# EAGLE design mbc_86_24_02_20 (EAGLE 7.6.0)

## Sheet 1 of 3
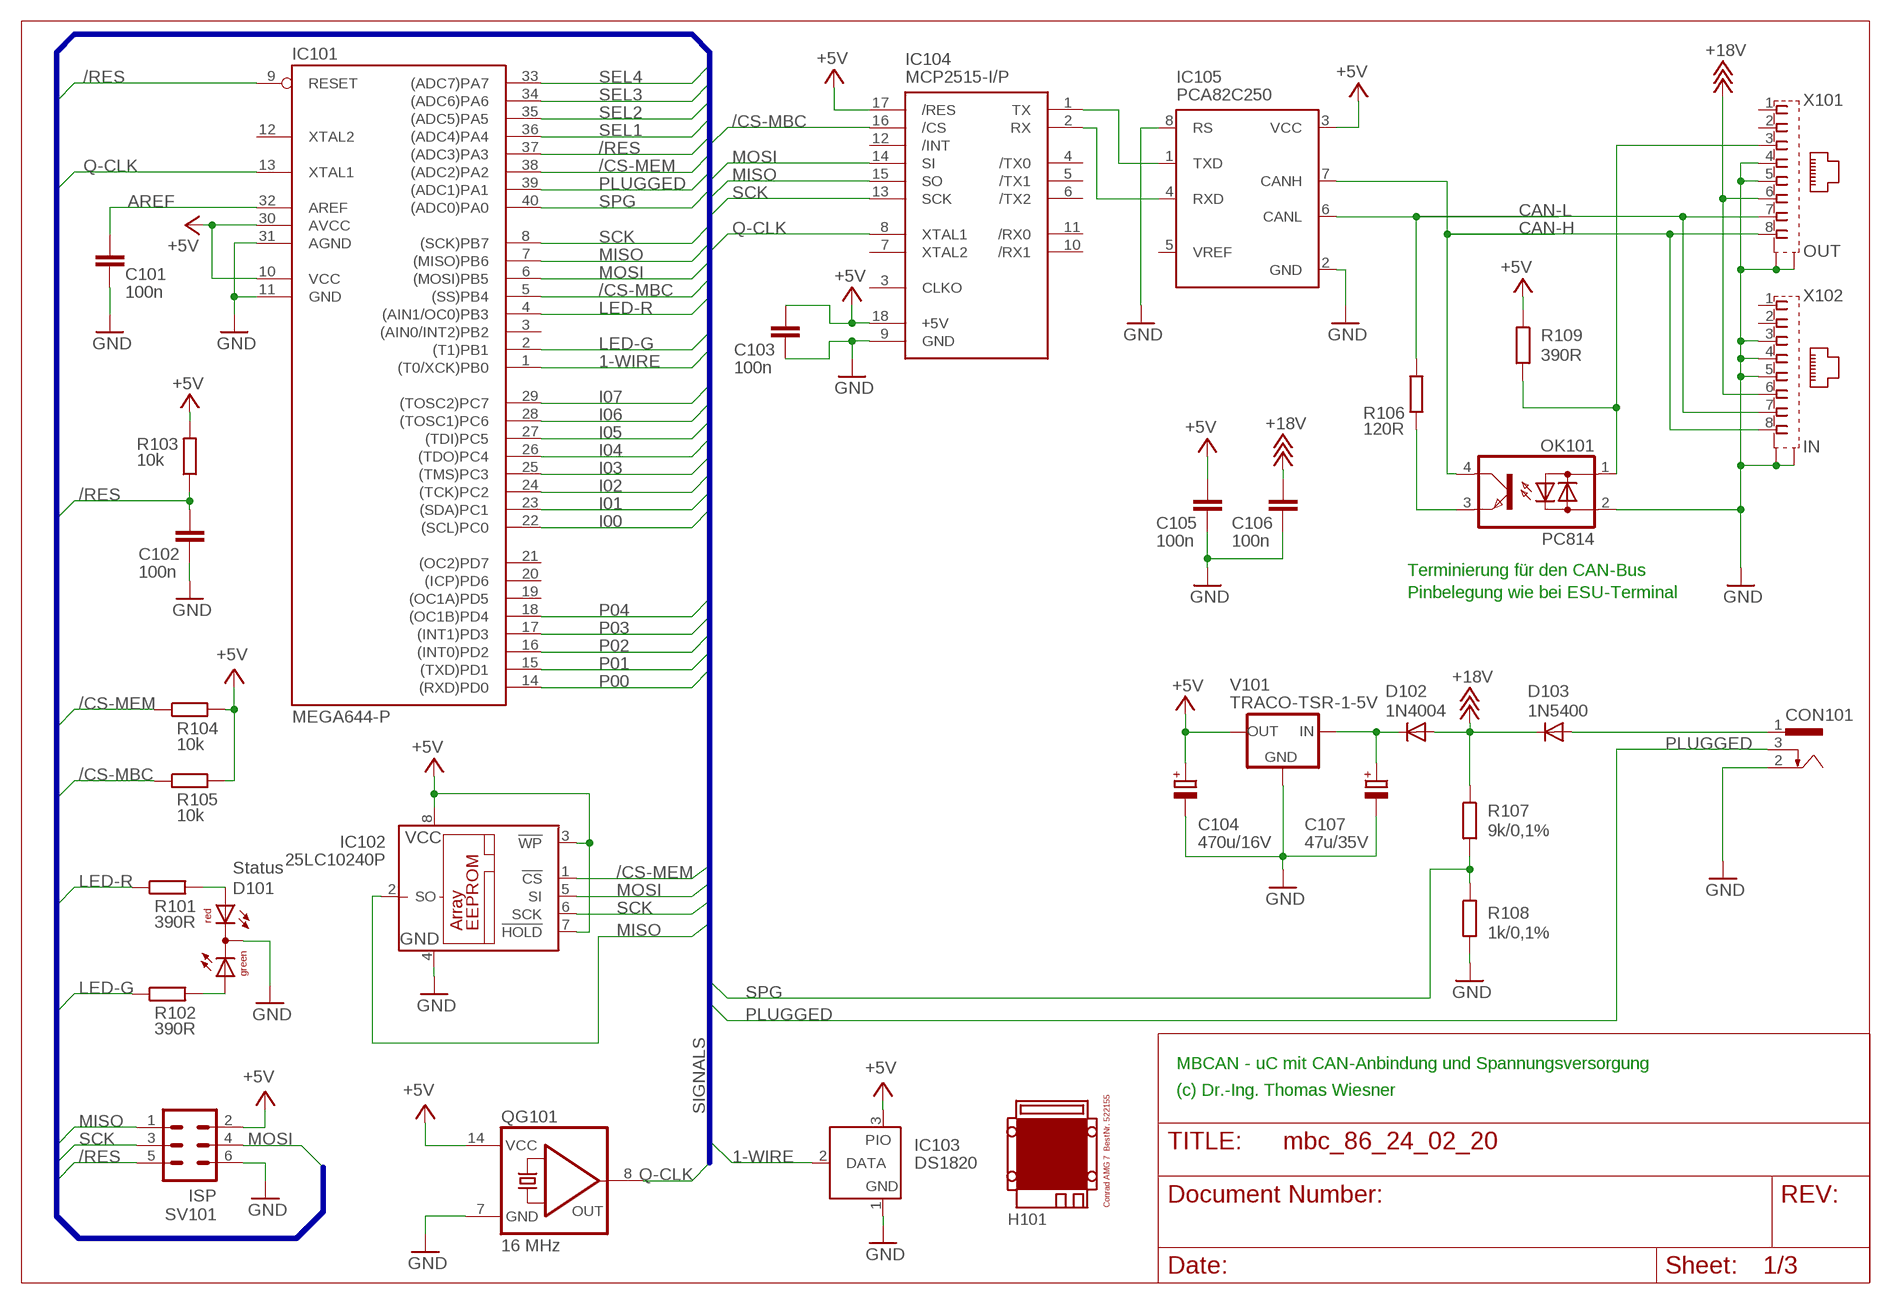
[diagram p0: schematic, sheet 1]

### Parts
C101  100n  C-EU025-025X050  [C025-025X050]
C102  100n  C-EU025-025X050  [C025-025X050]
C103  100n  C-EU025-025X050  [C025-025X050]
C104  470u/16V  CPOL-EUE3.5-8  [E3,5-8]
C105  100n  C-EU025-025X050  [C025-025X050]
C106  100n  C-EU025-025X050  [C025-025X050]
C107  47u/35V  CPOL-EUE2.5-7  [E2,5-7]
CON101  POWER-JACK  [POWER-JACK]
D101  Status  DUOLED5MM  [DUOLED5MM]
D102  1N4004  [DO41-10]
D103  1N5400  [DO201-15]
H101  MODULGEHÄUSE-AMG-7  [MODULGEHÄUSE-AMG-7]
IC101  MEGA644-P  MEGA323-P  [DIL40]
IC102  25LC10240P  25LC040P  [DIL8]
IC103  DS1820  DS2405  [TO92-]
IC104  MCP2515-I/P  MCP2510-I/P  [DIL18]
IC105  PCA82C250  [DIL08]
OK101  PC814  [DIL04]
QG101  16 MHz  QG5860  [DIL14S]
R101  390R  R-EU_0207/10  [0207/10]
R102  390R  R-EU_0207/10  [0207/10]
R103  10k  R-EU_0207/10  [0207/10]
R104  10k  R-EU_0207/10  [0207/10]
R105  10k  R-EU_0207/10  [0207/10]
R106  120R  R-EU_0207/10  [0207/10]
R107  9k/0,1%  R-EU_0207/10  [0207/10]
R108  1k/0,1%  R-EU_0207/10  [0207/10]
R109  390R  R-EU_0207/10  [0207/10]
SV101  ISP  ML6  [ML6]
V101  TRACO-TSR-1-5V  [TRACO-TSR-1]
X101  OUT  0446200002  [0446200002]
X102  IN  0446200002  [0446200002]

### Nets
1-WIRE: IC101.1((T0/XCK)PB0) IC103.2(DATA)
+5V: C103.1 C104.+ C105.1 IC101.10(VCC) IC101.30(AVCC) IC102.3(!WP) IC102.7(!HOLD) IC102.8(VCC) IC103.3(PIO) IC104.17(/RES) IC104.18(+5V) IC105.3(VCC) QG101.14(VCC) R103.2 R104.2 R105.2 R109.1 SV101.2 V101.OUT ; also sheet 2,3
+18V: C106.1 D102.A D103.C R107.1 X101.6 X102.6 ; also sheet 2
/CS-MBC: IC101.5((SS)PB4) IC104.16(/CS) R105.1
/CS-MEM: IC101.38((ADC2)PA2) IC102.1(!CS) R104.1
/RES: C102.1 IC101.9(RESET) IC101.37((ADC3)PA3) R103.1 SV101.5
AREF: C101.1 IC101.32(AREF)
CAN-H: IC105.7(CANH) OK101.4(C) X101.8 X102.8
CAN-L: IC105.6(CANL) R106.2 X101.7 X102.7
GND: C101.2 C102.2 C103.2 C104.- C105.2 C106.2 C107.- CON101.2 D101.K(C) IC101.11(GND) IC101.31(AGND) IC102.4(GND) IC103.1(GND) IC104.9(GND) IC105.2(GND) IC105.8(RS) OK101.2(AC2) QG101.7(GND) R108.2 SV101.6 V101.GND X101.4 X101.5 X101.S@1(S1) X101.S@2(S2) X102.3 X102.4 X102.5 X102.S@1(S1) X102.S@2(S2) ; also sheet 2,3
I00: IC101.22((SCL)PC0) ; also sheet 3
I01: IC101.23((SDA)PC1) ; also sheet 3
I02: IC101.24((TCK)PC2) ; also sheet 3
I03: IC101.25((TMS)PC3) ; also sheet 3
I04: IC101.26((TDO)PC4) ; also sheet 3
I05: IC101.27((TDI)PC5) ; also sheet 3
I06: IC101.28((TOSC1)PC6) ; also sheet 3
I07: IC101.29((TOSC2)PC7) ; also sheet 3
LED-G: IC101.2((T1)PB1) R102.1
LED-R: IC101.4((AIN1/OC0)PB3) R101.1
MISO: IC101.7((MISO)PB6) IC102.2(SO) IC104.15(SO) SV101.1
MOSI: IC101.6((MOSI)PB5) IC102.5(SI) IC104.14(SI) SV101.4
N$1: IC104.1(TX) IC105.1(TXD)
N$2: IC104.2(RX) IC105.4(RXD)
N$3: OK101.3(E) R106.1
N$5: OK101.1(AC1) R109.2 X101.3
N$6: C107.+ D102.C V101.IN
N$9: D101.AR R101.2
N$13: D101.AG R102.2
P00: IC101.14((RXD)PD0) ; also sheet 2
P01: IC101.15((TXD)PD1) ; also sheet 2
P02: IC101.16((INT0)PD2) ; also sheet 2
P03: IC101.17((INT1)PD3) ; also sheet 2
P04: IC101.18((OC1B)PD4) ; also sheet 2
PLUGGED: CON101.3 IC101.39((ADC1)PA1)
Q-CLK: IC101.13(XTAL1) IC104.8(XTAL1) QG101.8(OUT)
SCK: IC101.8((SCK)PB7) IC102.6(SCK) IC104.13(SCK) SV101.3
SEL1: IC101.36((ADC4)PA4) ; also sheet 2
SEL2: IC101.35((ADC5)PA5) ; also sheet 2
SEL3: IC101.34((ADC6)PA6)
SEL4: IC101.33((ADC7)PA7)
SPG: IC101.40((ADC0)PA0) R107.2 R108.1
V-NETZTEIL1: CON101.1 D103.A
Unconnected: IC101.3((AIN0/INT2)PB2) IC101.12(XTAL2) IC101.19((OC1A)PD5) IC101.20((ICP)PD6) IC101.21((OC2)PD7) IC104.3(CLKO) IC104.4(/TX0) IC104.5(/TX1) IC104.6(/TX2) IC104.7(XTAL2) IC104.10(/RX1) IC104.11(/RX0) IC104.12(/INT) IC105.5(VREF) X101.1 X101.2 X102.1 X102.2

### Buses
SIGNALS

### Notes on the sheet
- Terminierung für den CAN-Bus
- Pinbelegung wie bei ESU-Terminal
- MBCAN - uC mit CAN-Anbindung und Spannungsversorgung
- (c) Dr.-Ing. Thomas Wiesner

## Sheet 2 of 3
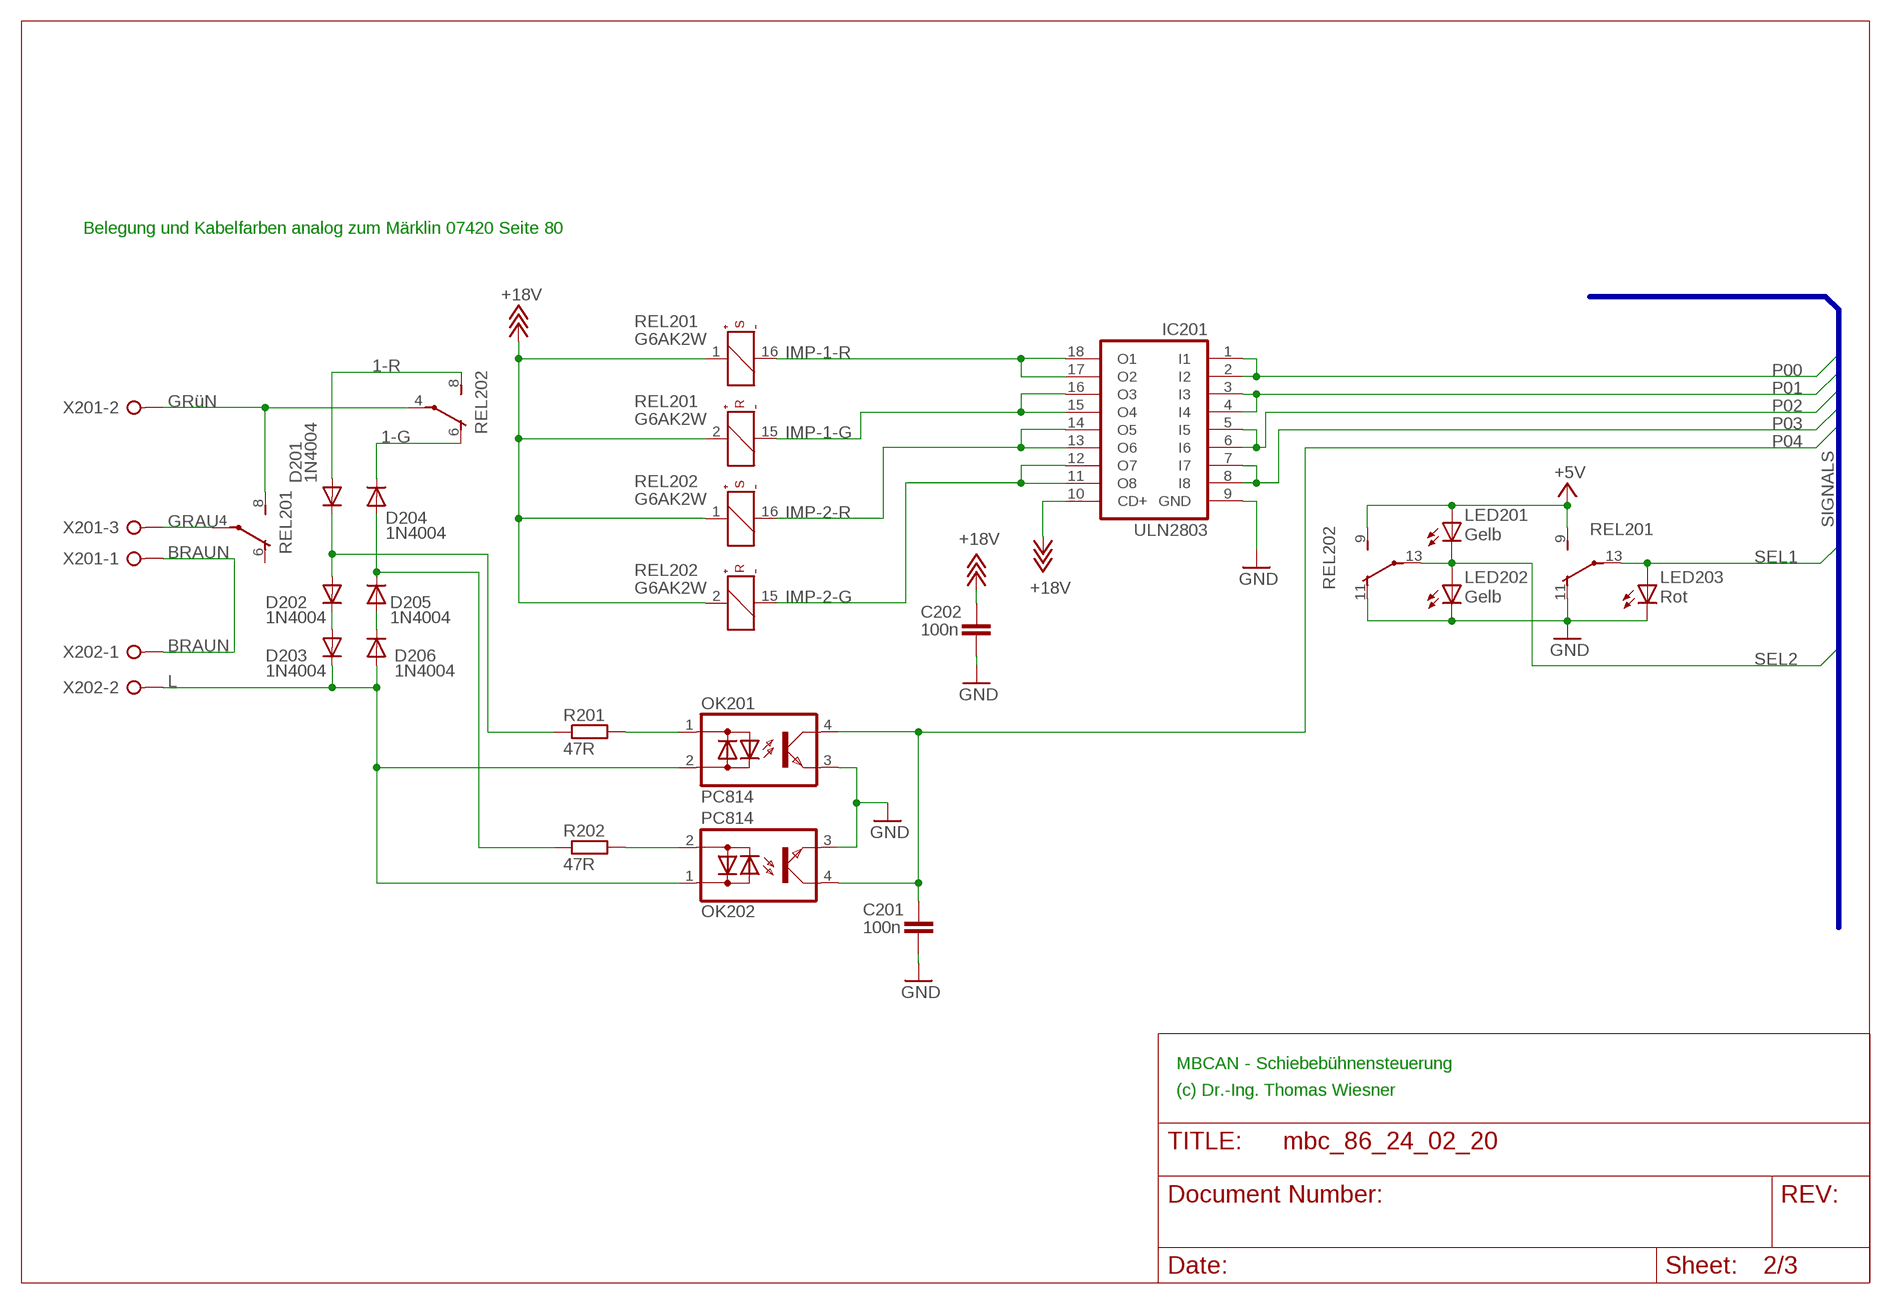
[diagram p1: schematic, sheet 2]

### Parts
C201  100n  C-EU025-025X050  [C025-025X050]
C202  100n  C-EU025-025X050  [C025-025X050]
D201  1N4004  [DO41-10]
D202  1N4004  [DO41-10]
D203  1N4004  [DO41-10]
D204  1N4004  [DO41-10]
D205  1N4004  [DO41-10]
D206  1N4004  [DO41-10]
IC201  ULN2803  ULN2803A  [DIL18]
LED201  Gelb  LED3MM  [LED3MM]
LED202  Gelb  LED3MM  [LED3MM]
LED203  Rot  LED3MM  [LED3MM]
OK201  PC814  [DIL04]
OK202  PC814  [DIL04]
R201  47R  R-EU_0207/10  [0207/10]
R202  47R  R-EU_0207/10  [0207/10]
REL201  G6AK2W  [REL-BIPOLAR]
REL202  G6AK2W  [REL-BIPOLAR]
X201  W237-03P  [W237-133]
X202  W237-02P  [W237-132]

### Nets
1-G: D204.C REL202.6(O)
1-R: D201.A REL202.8(S)
+5V: LED201.A REL201.9(S) REL202.9(S) ; also sheet 1,3
+18V: C202.1 IC201.10(CD+) REL201.1(+) REL201.2(+) REL202.1(+) REL202.2(+) ; also sheet 1
BRAUN: X201.1 X202.1
GND: C201.2 C202.2 IC201.9(GND) LED202.K(C) LED203.K(C) OK201.3(E) OK202.3(E) REL201.11(O) REL202.11(O) ; also sheet 1,3
GRAU: REL201.4(P) X201.3
GRüN: REL201.8(S) REL202.4(P) X201.2
IMP-1-G: IC201.15(O4) IC201.16(O3) REL201.15(-)
IMP-1-R: IC201.17(O2) IC201.18(O1) REL201.16(-)
IMP-2-G: IC201.11(O8) IC201.12(O7) REL202.15(-)
IMP-2-R: IC201.13(O6) IC201.14(O5) REL202.16(-)
L: D203.C D206.A OK201.2(AC2) OK202.1(AC1) X202.2
N$4: D202.C D203.A
N$7: D205.A D206.C
N$8: OK202.2(AC2) R202.2
N$10: OK201.1(AC1) R201.2
P00: IC201.1(I1) IC201.2(I2) ; also sheet 1
P01: IC201.3(I3) IC201.4(I4) ; also sheet 1
P02: IC201.5(I5) IC201.6(I6) ; also sheet 1
P03: IC201.7(I7) IC201.8(I8) ; also sheet 1
P04: C201.1 OK201.4(C) OK202.4(C) ; also sheet 1
SCH-1-G: D204.A D205.C R202.1
SCH-1-R: D201.C D202.A R201.1
SEL1: LED203.A REL201.13(P) ; also sheet 1
SEL2: LED201.K(C) LED202.A REL202.13(P) ; also sheet 1
Unconnected: REL201.6(O)

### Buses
SIGNALS

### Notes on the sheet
- Belegung und Kabelfarben analog zum Märklin 07420 Seite 80
- MBCAN - Schiebebühnensteuerung
- (c) Dr.-Ing. Thomas Wiesner

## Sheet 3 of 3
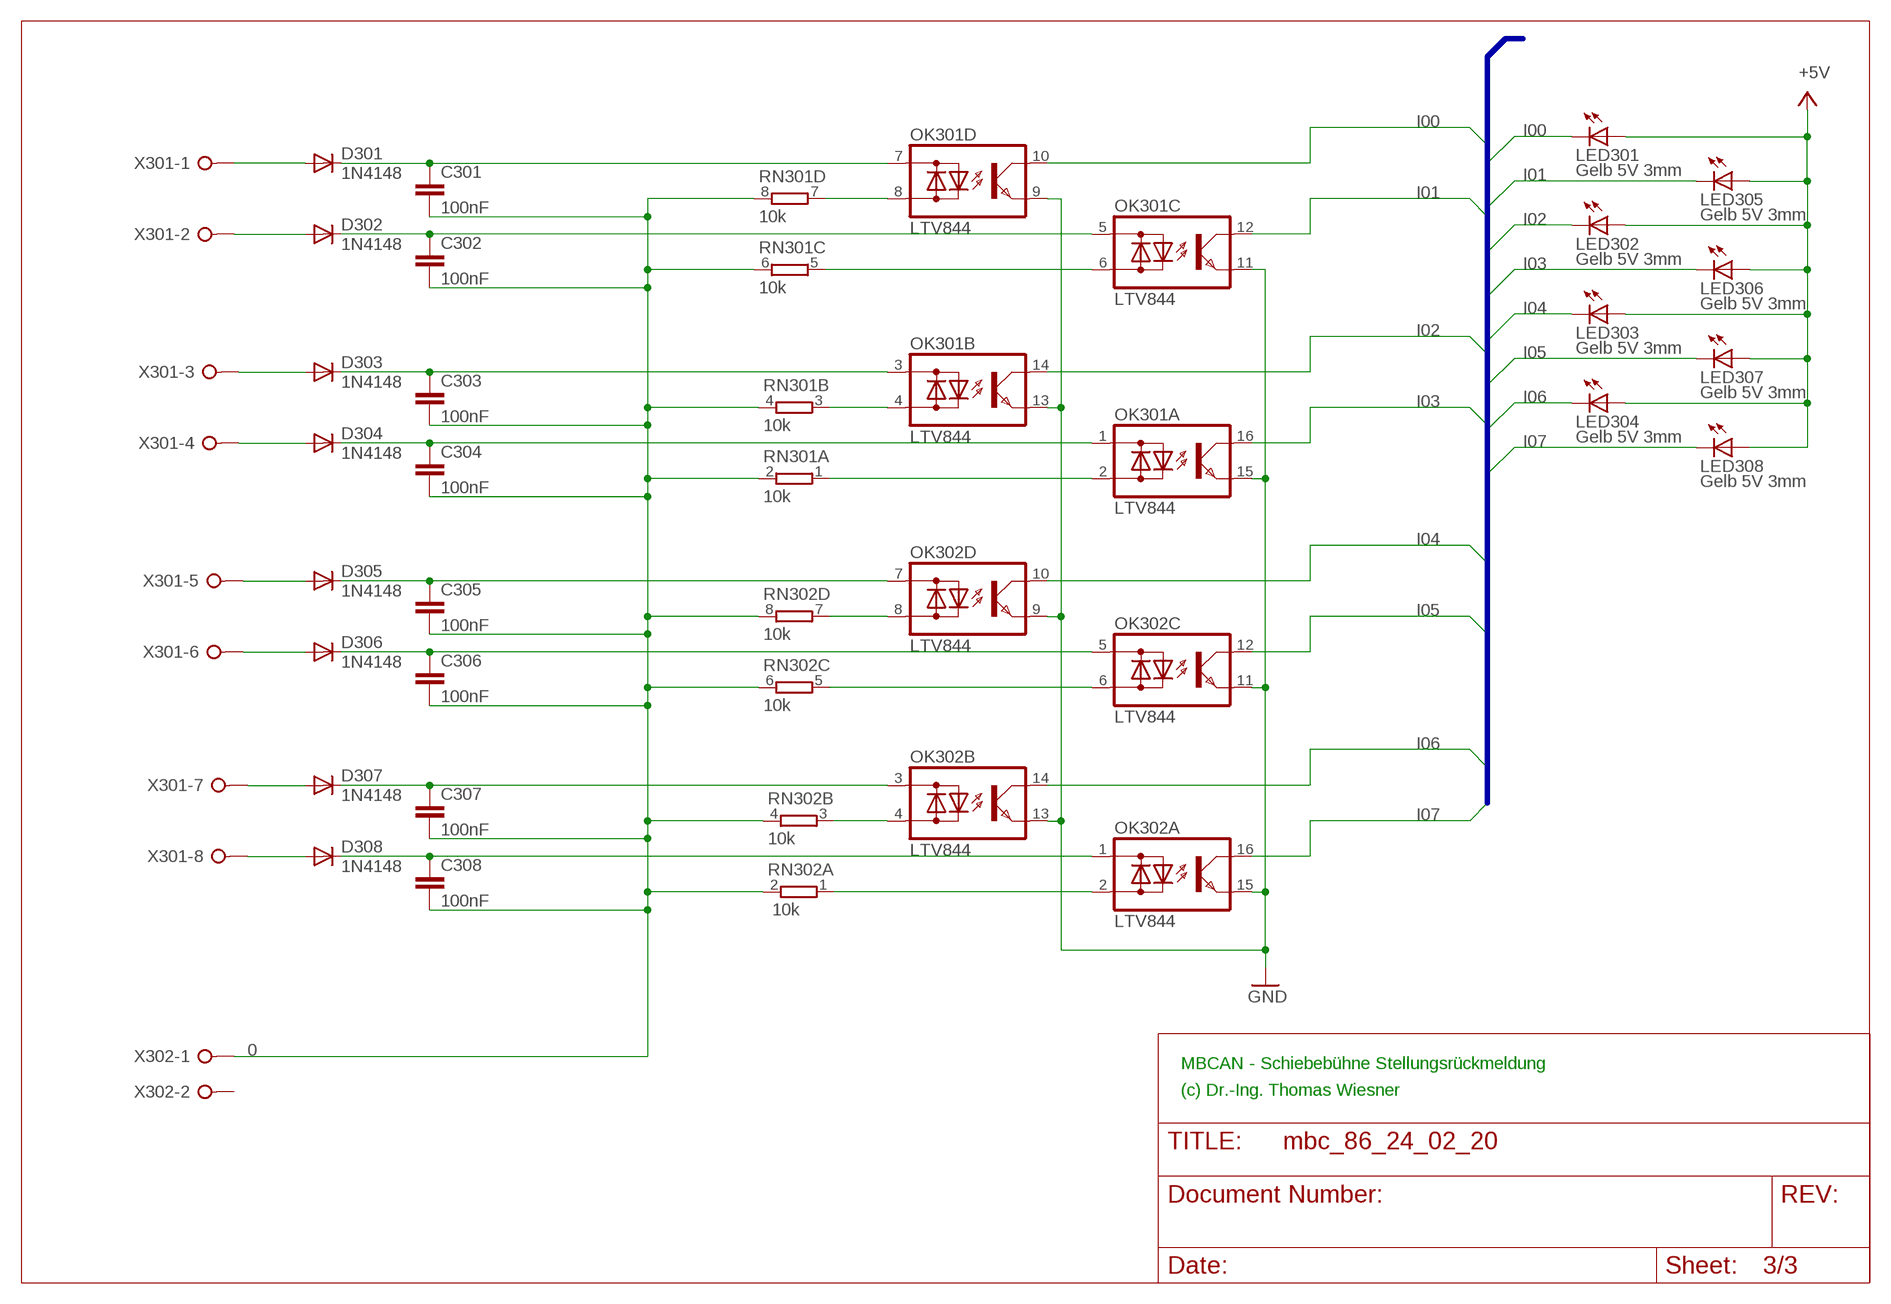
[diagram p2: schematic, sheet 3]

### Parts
C301  100nF  C-EU025-025X050  [C025-025X050]
C302  100nF  C-EU025-025X050  [C025-025X050]
C303  100nF  C-EU025-025X050  [C025-025X050]
C304  100nF  C-EU025-025X050  [C025-025X050]
C305  100nF  C-EU025-025X050  [C025-025X050]
C306  100nF  C-EU025-025X050  [C025-025X050]
C307  100nF  C-EU025-025X050  [C025-025X050]
C308  100nF  C-EU025-025X050  [C025-025X050]
D301  1N4148  1N4148DO35-10  [DO35-10]
D302  1N4148  1N4148DO35-10  [DO35-10]
D303  1N4148  1N4148DO35-10  [DO35-10]
D304  1N4148  1N4148DO35-10  [DO35-10]
D305  1N4148  1N4148DO35-10  [DO35-10]
D306  1N4148  1N4148DO35-10  [DO35-10]
D307  1N4148  1N4148DO35-10  [DO35-10]
D308  1N4148  1N4148DO35-10  [DO35-10]
LED301  Gelb 5V 3mm  LED3MM  [LED3MM]
LED302  Gelb 5V 3mm  LED3MM  [LED3MM]
LED303  Gelb 5V 3mm  LED3MM  [LED3MM]
LED304  Gelb 5V 3mm  LED3MM  [LED3MM]
LED305  Gelb 5V 3mm  LED3MM  [LED3MM]
LED306  Gelb 5V 3mm  LED3MM  [LED3MM]
LED307  Gelb 5V 3mm  LED3MM  [LED3MM]
LED308  Gelb 5V 3mm  LED3MM  [LED3MM]
OK301  LTV844  TIL196  [DIL16]
OK302  LTV844  TIL196  [DIL16]
RN301  10k  E4R  [SIL8]
RN302  10k  E4R  [SIL8]
X301  W237-08P  [W237-8P]
X302  W237-02P  [W237-132]

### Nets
0: C301.2 C302.2 C303.2 C304.2 C305.2 C306.2 C307.2 C308.2 RN301.2 RN301.4 RN301.6 RN301.8 RN302.2 RN302.4 RN302.6 RN302.8 X302.1
+5V: LED301.A LED302.A LED303.A LED304.A LED305.A LED306.A LED307.A LED308.A ; also sheet 1,2
GND: OK301.9(D:E) OK301.11(C:E) OK301.13(B:E) OK301.15(A:E) OK302.9(D:E) OK302.11(C:E) OK302.13(B:E) OK302.15(A:E) ; also sheet 1,2
I00: LED301.K(C) OK301.10(D:C) ; also sheet 1
I01: LED305.K(C) OK301.12(C:C) ; also sheet 1
I02: LED302.K(C) OK301.14(B:C) ; also sheet 1
I03: LED306.K(C) OK301.16(A:C) ; also sheet 1
I04: LED303.K(C) OK302.10(D:C) ; also sheet 1
I05: LED307.K(C) OK302.12(C:C) ; also sheet 1
I06: LED304.K(C) OK302.14(B:C) ; also sheet 1
I07: LED308.K(C) OK302.16(A:C) ; also sheet 1
N$11: D301.A X301.1
N$12: C301.1 D301.C OK301.7(D:AC1)
N$14: C302.1 D302.C OK301.5(C:AC1)
N$15: C303.1 D303.C OK301.3(B:AC1)
N$16: D302.A X301.2
N$17: D303.A X301.3
N$18: C304.1 D304.C OK301.1(A:AC1)
N$19: D304.A X301.4
N$20: C305.1 D305.C OK302.7(D:AC1)
N$21: C306.1 D306.C OK302.5(C:AC1)
N$22: C307.1 D307.C OK302.3(B:AC1)
N$23: C308.1 D308.C OK302.1(A:AC1)
N$24: D305.A X301.5
N$25: D306.A X301.6
N$26: D308.A X301.8
N$27: D307.A X301.7
N$42: OK302.2(A:AC2) RN302.1
N$43: OK302.4(B:AC2) RN302.3
N$44: OK302.6(C:AC2) RN302.5
N$45: OK302.8(D:AC2) RN302.7
N$46: OK301.2(A:AC2) RN301.1
N$48: OK301.4(B:AC2) RN301.3
N$64: OK301.6(C:AC2) RN301.5
N$65: OK301.8(D:AC2) RN301.7
Unconnected: X302.2

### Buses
B$1

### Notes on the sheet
- MBCAN - Schiebebühne Stellungsrückmeldung
- (c) Dr.-Ing. Thomas Wiesner

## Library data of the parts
C101-C103 C105 C106 C201 C202 C301-C308 = rcl:C-EU: CAPACITOR, European symbol
C104 C107 = rcl:CPOL-EU: POLARIZED CAPACITOR, European symbol
CON101 = mbc:POWER-JACK: Power-Stecker für 2,5 mm Hohlbuchse
D101 = led:DUOLED5MM: DUO LED 2 colors, 5 mm, round
D102 D201-D206 = diode:1N4004: DIODE
D103 = diode:1N5400: DIODE
D301-D308 = diode:1N4148: DIODE
H101 = mbc:MODULGEHÄUSE-AMG-7: Gehäuse
IC101 = atmel:MEGA323-P: MICROCONTROLLER 32 Kbytes FLASH 2 Kbytes SRAM 1 Kbytes EEPROM USART 8-channel 10 bit ADC Source: avr.lbr; OC_FARNELL: unknown; OC_NEWARK: unknown
IC102 = microchip:25*: Serial EEPROM 4K/ 8K , SPI bus; MF: MICROCHIP; MPN: 25LC040/P; OC_FARNELL: 9758100; OC_NEWARK: 96K4091
IC103 = maxim:DS2405: Addressable Switch DALLAS Semiconductor; MF: DALLAS SEMICONDUCTOR; MPN: DS2405; OC_FARNELL: 1188025; OC_NEWARK: 06F4645
IC104 = mbc:MCP2510: BASIC-CAN 2.0a Controller Stand-alone CAN controller von Microchip
IC105 = micro-philips:PCA82C250: CAN CONTROLLER INTERFACE; OC_FARNELL: 3692358; OC_NEWARK: unknown
IC201 = uln-udn:ULN2803A: DRIVER ARRAY
LED201-LED203 LED301-LED308 = led:LED: LED
OK101 OK201 OK202 = optocoupler:PC814: SHARP OPTO COUPLER; OC_FARNELL: 9707662; OC_NEWARK: unknown
OK301 OK302 = optocoupler:TIL196: TEXAS INSTRUMENTS OPTO COUPLER; MPN: TIL 196; OC_FARNELL: 1683367; OC_NEWARK: 05R6476
QG101 = crystal:QG5860: CRYSTAL RESONATOR; OC_FARNELL: unknown; OC_NEWARK: unknown
R101-R109 = resistor:R-EU_: RESISTOR, European symbol
R201 R202 = rcl:R-EU_: RESISTOR, European symbol
REL201 REL202 = mbc:G6AK2W: Bipolares Relais 2xUM 12V
RN301 RN302 = resistor-sil:E4R: SIL RESISTOR; OC_FARNELL: unknown; OC_NEWARK: unknown
SV101 = con-ml:ML6: HARTING; OC_FARNELL: unknown; OC_NEWARK: unknown
V101 = mbc:TRACO-TSR-1-5V: Spannungsregler Hersteller: TRACO Typ: TSR-1 5V: TSR 1-2450 Spg: 5V Strom: 1A Reichelt TSR 1-2450
X101 X102 = mbc:0446200002: RJ-45 INVERTED MODULAR JACK ASSEMBLY WITH RJ-11 KEEPOUT FEATURE Source: Data sheet MOLEX 0446200002 BUCHSE, RJ45, GESCHIRMT Source: Farnell; MF: MOLEX; MPN: 0446200002; OC_FARNELL: 9251910
X201 = con-wago-508:W237-03P: WAGO SREW CLAMP; OC_FARNELL: unknown; OC_NEWARK: unknown
X202 X302 = con-wago-508:W237-02P: WAGO SREW CLAMP; OC_FARNELL: unknown; OC_NEWARK: unknown
X301 = con-wago-508:W237-08P: WAGO SREW CLAMP; OC_FARNELL: unknown; OC_NEWARK: unknown

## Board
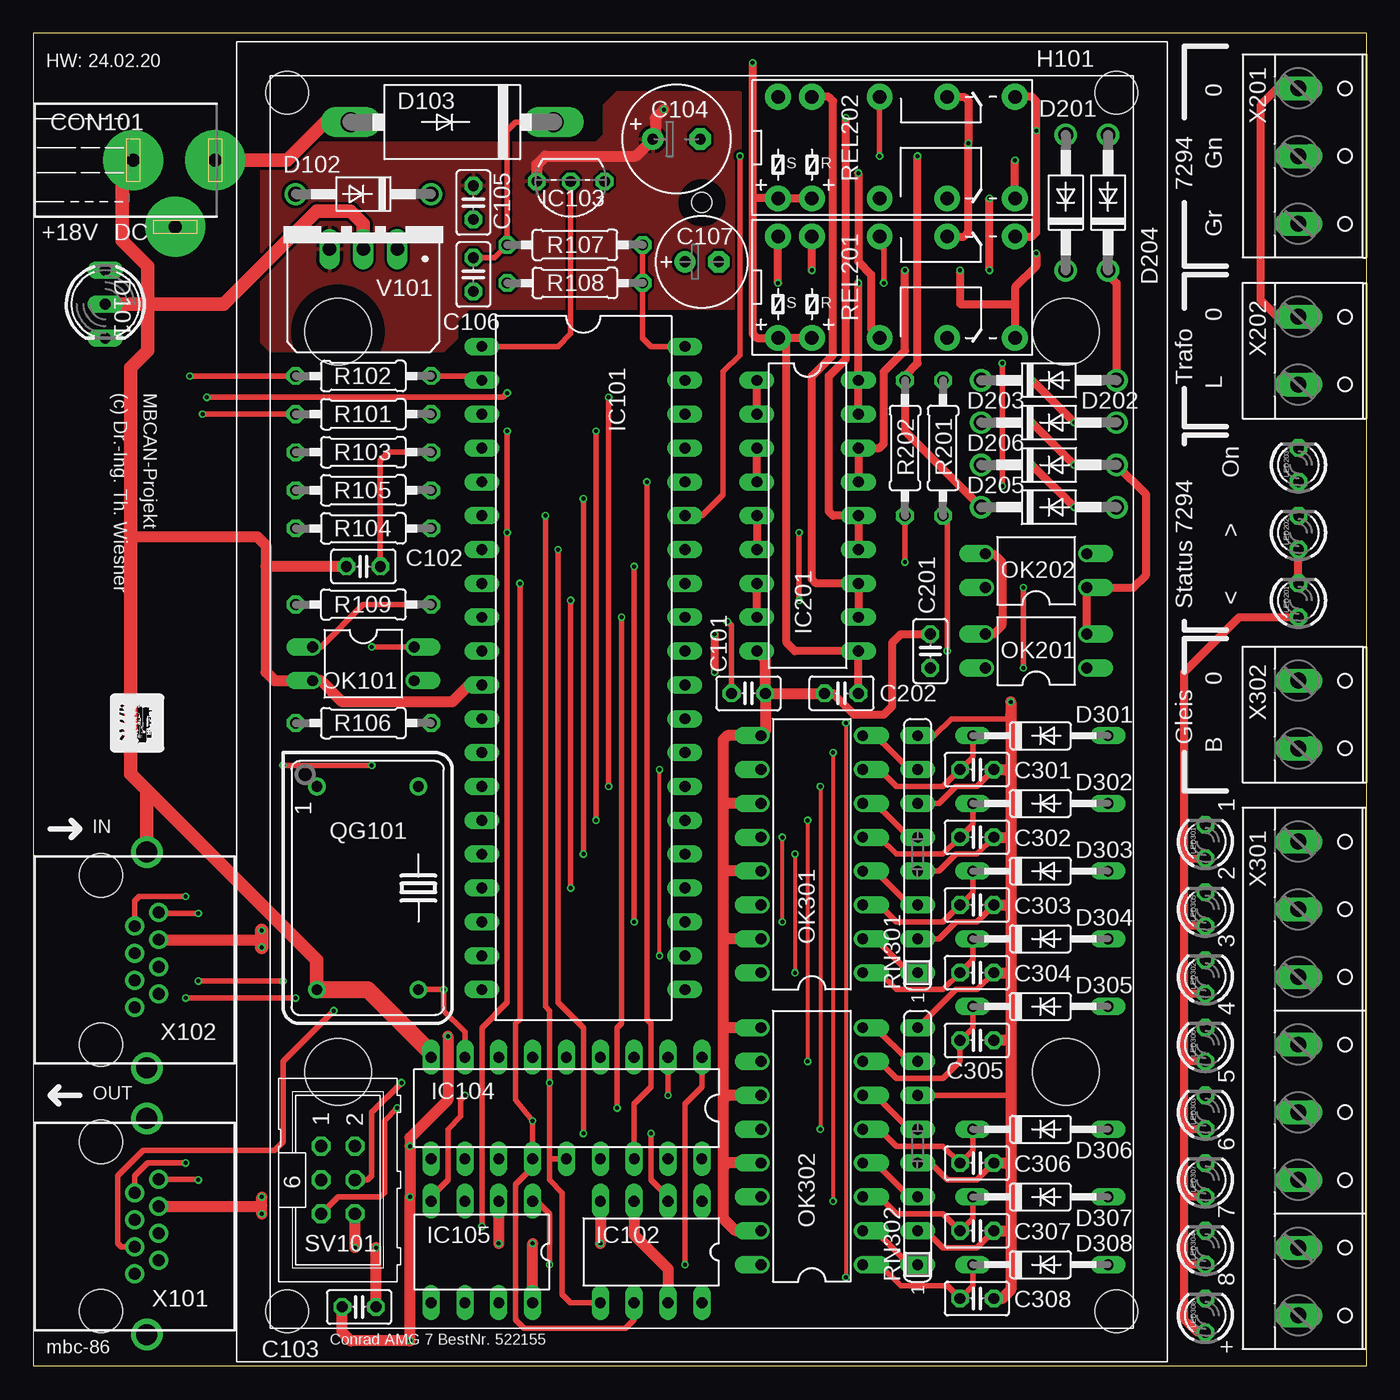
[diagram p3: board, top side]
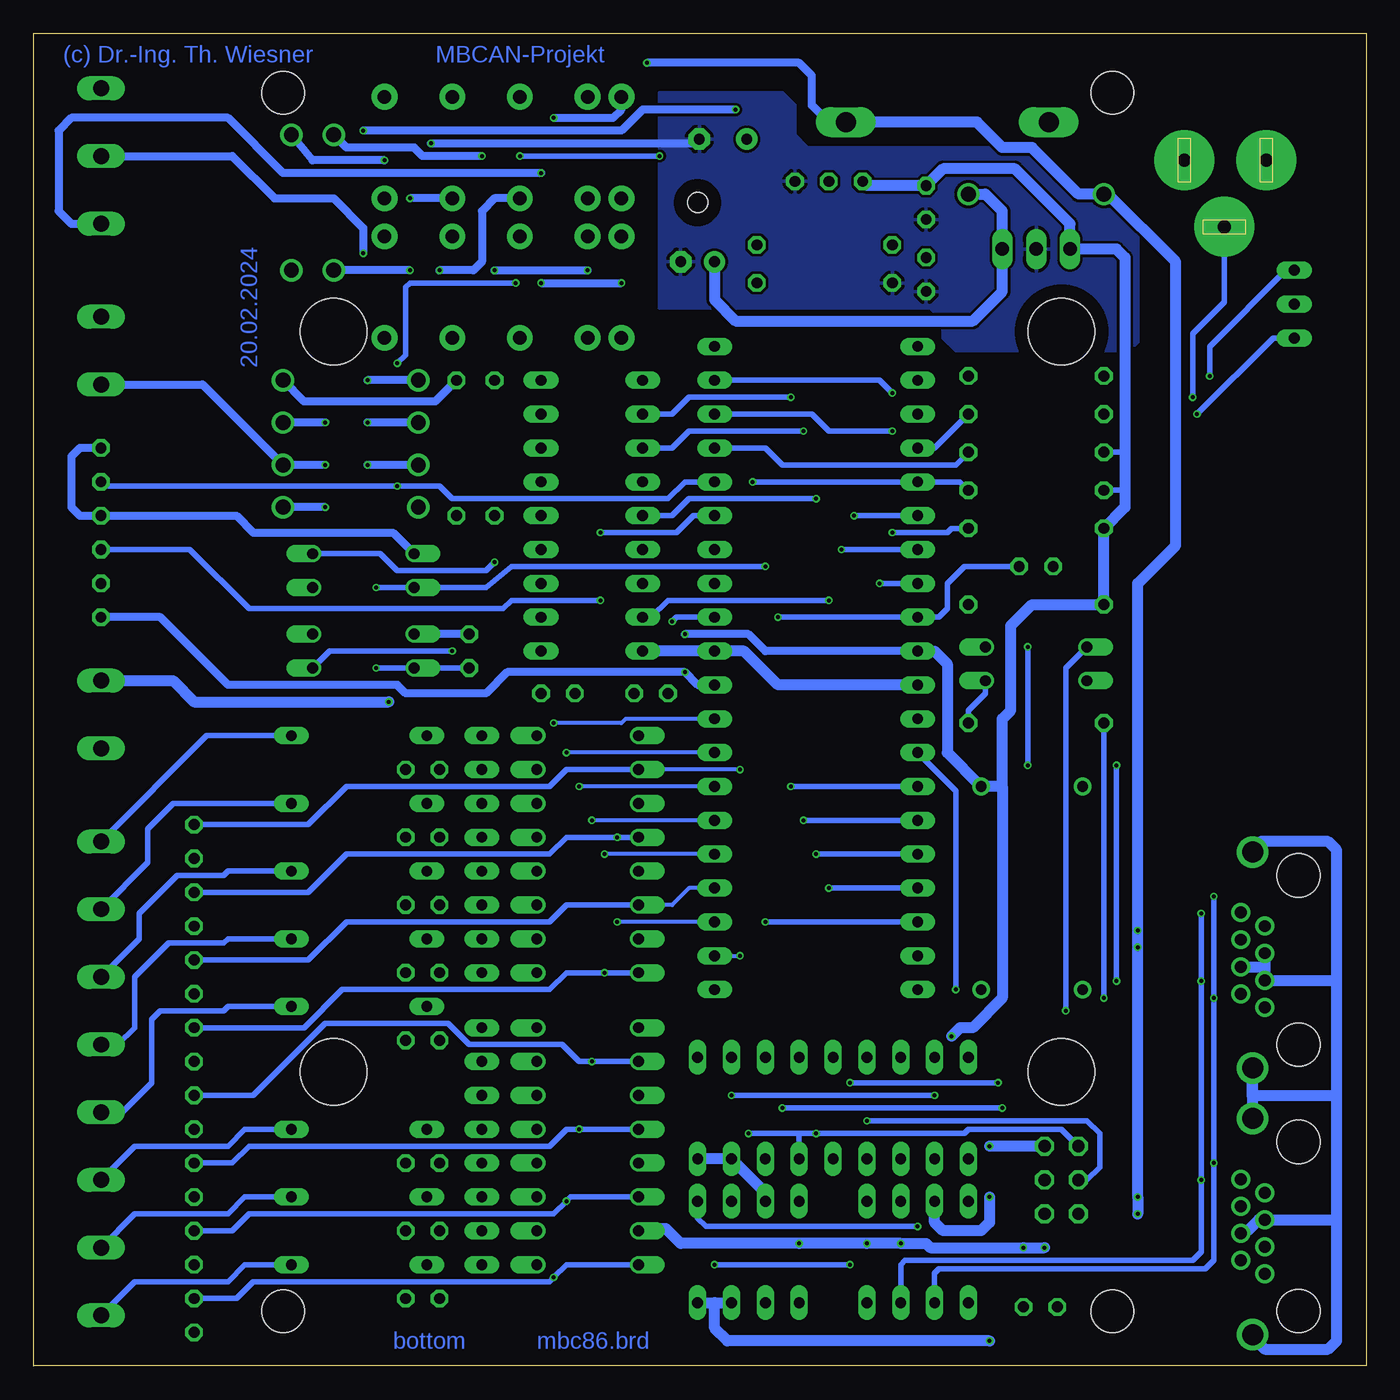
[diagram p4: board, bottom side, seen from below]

Size 100.01 x 100.01 mm. Coordinates in mm from the lower left corner, seen from the top.
Outline: 100,0.02 0,0.02 0,100.01 100,100.01
Outline: 100.01,100.01 100.01,0
Copper layers (1*16): Top 0.035mm / dielectric 1.5mm / Bottom 0.035mm
Design rules "default *": minimum track width 10mil, minimum drill 0.3mm, track to track 8mil, track to pad 8mil, pad to pad 8mil, via to via 8mil, smd to smd 8mil, copper to edge 40mil, drill to drill 8mil, minimum pad ring 10mil, minimum via ring 0.125mm, stop-mask expansion 4mil, vias tented up to drill 0mil, thermal gap 10mil

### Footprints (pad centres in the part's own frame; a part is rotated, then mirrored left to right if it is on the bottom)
C025-025X050 = drill 0.813 octagon: 1 -1.27,0; 2 1.27,0
E3,5-8 = drill 0.813 pad 1.6: + -1.778,0 | drill 0.813 pad 1.6 octagon: - 1.778,0
E2,5-7 = drill 0.813 pad 1.6: + -1.27,0 | drill 0.813 pad 1.6 octagon: - 1.27,0
POWER-JACK = drill 1 pad 4.5: 1 0,6.03; 2 0,-0.12; 3 5,3.03
DUOLED5MM = drill 0.813 long: AG -2.54,0; AR 2.54,0; K 0,0
DO41-10 = drill 1.118: A 5.08,0; C -5.08,0
DO201-15 = drill 1.499 long: A 7.62,0; C -7.62,0
DO35-10 = drill 0.813 long: A 5.08,0; C -5.08,0
MODULGEHÄUSE-AMG-7 = hole 3.2: -45.72,-31.115; -45.72,31.115; 45.72,31.115; 45.72,-31.115 | hole 5: -27.781,-27.305; 27.781,-27.305; -27.781,27.305; 27.781,27.305 | hole 1.5: -37.465,0
DIL40 = drill 0.813 long: 1 -24.13,-7.62; 2 -21.59,-7.62; 3 -19.05,-7.62; 4 -16.51,-7.62; 5 -13.97,-7.62; 6 -11.43,-7.62; 7 -8.89,-7.62; 8 -6.35,-7.62; 9 -3.81,-7.62; 10 -1.27,-7.62; 11 1.27,-7.62; 12 3.81,-7.62; 13 6.35,-7.62; 14 8.89,-7.62; 15 11.43,-7.62; 16 13.97,-7.62; 17 16.51,-7.62; 18 19.05,-7.62; 19 21.59,-7.62; 20 24.13,-7.62; 21 24.13,7.62; 22 21.59,7.62; 23 19.05,7.62; 24 16.51,7.62; 25 13.97,7.62; 26 11.43,7.62; 27 8.89,7.62; 28 6.35,7.62; 29 3.81,7.62; 30 1.27,7.62; 31 -1.27,7.62; 32 -3.81,7.62; 33 -6.35,7.62; 34 -8.89,7.62; 35 -11.43,7.62; 36 -13.97,7.62; 37 -16.51,7.62; 38 -19.05,7.62; 39 -21.59,7.62; 40 -24.13,7.62
DIL8 = drill 0.813 long: 1 -3.81,-3.81; 2 -1.27,-3.81; 3 1.27,-3.81; 4 3.81,-3.81; 5 3.81,3.81; 6 1.27,3.81; 7 -1.27,3.81; 8 -3.81,3.81
TO92- = drill 0.813 octagon: 1 -2.54,0; 2 0,0; 3 2.54,0
DIL18 = drill 0.813 long: 1 -10.16,-3.81; 2 -7.62,-3.81; 3 -5.08,-3.81; 4 -2.54,-3.81 | drill 0.8 long: 5 0,-3.81; 6 2.54,-3.81; 7 5.08,-3.81; 8 7.62,-3.81; 9 10.16,-3.81; 10 10.16,3.81; 11 7.62,3.81; 12 5.08,3.81; 13 2.54,3.81; 14 0,3.81; 15 -2.54,3.81; 16 -5.08,3.81; 17 -7.62,3.81; 18 -10.16,3.81
DIL08 = drill 0.813 long: 1 -3.81,-3.81; 2 -1.27,-3.81; 3 1.27,-3.81; 4 3.81,-3.81; 5 3.81,3.81; 6 1.27,3.81; 7 -1.27,3.81; 8 -3.81,3.81
DIL18' = drill 0.813 long: 1 -10.16,-3.81; 2 -7.62,-3.81; 3 -5.08,-3.81; 4 -2.54,-3.81; 5 0,-3.81; 6 2.54,-3.81; 7 5.08,-3.81; 8 7.62,-3.81; 9 10.16,-3.81; 10 10.16,3.81; 11 7.62,3.81; 12 5.08,3.81; 13 2.54,3.81; 14 0,3.81; 15 -2.54,3.81; 16 -5.08,3.81; 17 -7.62,3.81; 18 -10.16,3.81
LED3MM = drill 0.813 octagon: A -1.27,0; K 1.27,0
DIL04 = drill 0.813 offset: 1 -1.27,-3.81; 2 1.27,-3.81; 3 1.27,3.81; 4 -1.27,3.81
DIL16 = drill 0.813 offset: 1 -8.89,-3.81; 2 -6.35,-3.81; 3 -3.81,-3.81; 4 -1.27,-3.81; 5 1.27,-3.81; 6 3.81,-3.81; 7 6.35,-3.81; 8 8.89,-3.81; 9 8.89,3.81; 10 6.35,3.81; 11 3.81,3.81; 12 1.27,3.81; 13 -1.27,3.81; 14 -3.81,3.81; 15 -6.35,3.81; 16 -8.89,3.81
DIL14S = drill 0.813: 1 -7.62,-3.81; 7 7.62,-3.81; 8 7.62,3.81; 14 -7.62,3.81
0207/10 = drill 0.813 octagon: 1 -5.08,0; 2 5.08,0
REL-BIPOLAR = drill 1.016 pad 1.93: 1 -8.89,-3.81; 2 -6.35,-3.81; 4 -1.27,-3.81; 6 3.81,-3.81; 8 8.89,-3.81; 9 8.89,3.81; 11 3.81,3.81; 13 -1.27,3.81; 15 -6.35,3.81; 16 -8.89,3.81
SIL8 = drill 0.813 long: 1 -8.89,0; 2 -6.35,0; 3 -3.81,0; 4 -1.27,0; 5 1.27,0; 6 3.81,0; 7 6.35,0; 8 8.89,0
ML6 = drill 0.914 octagon: 1 -2.54,-1.27; 2 -2.54,1.27; 3 0,-1.27; 4 0,1.27; 5 2.54,-1.27; 6 2.54,1.27
TRACO-TSR-1 = drill 1.016 long: GND 0,2.54; IN -2.54,2.54; OUT 2.54,2.54
0446200002 = drill 0.889 pad 1.422: 1 3.556,2.54; 2 2.54,4.318; 3 1.524,2.54; 4 0.508,4.318; 5 -0.508,2.54; 6 -1.524,4.318; 7 -2.54,2.54; 8 -3.556,4.318 | drill 1.575 pad 2.286: S@1 -8.103,3.429; S@2 8.103,3.429 | hole 3.251: 6.35,0; -6.35,0
W237-133 = drill 1.194 long: 1 -5.08,-0.635; 2 0,-0.635; 3 5.08,-0.635
W237-132 = drill 1.194 long: 1 -2.54,-0.635; 2 2.54,-0.635
W237-8P = drill 1.194 long: 1 -17.78,-0.635; 2 -12.7,-0.635; 3 -7.62,-0.635; 4 -2.54,-0.635; 5 2.54,-0.635; 6 7.62,-0.635; 7 12.7,-0.635; 8 17.78,-0.635

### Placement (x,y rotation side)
C101  53.66,50.48 0 top
C102  24.77,60.01 180 top
C103  24.45,4.45 0 top
C104  48.26,92.08 0 top
C105  33.02,87.31 270 top
C106  33.02,81.92 270 top
C107  50.16,82.87 0 top
C201  67.31,53.66 90 top
C202  60.64,50.48 180 top
C301  70.8,44.77 0 top
C302  70.8,39.69 0 top
C303  70.8,34.61 0 top
C304  70.8,29.53 0 top
C305  70.8,24.45 0 top
C306  70.8,15.24 0 top
C307  70.8,10.16 0 top
C308  70.8,5.08 0 top
CON101  7.62,90.49 270 top
D101  5.4,79.69 270 top
D102  24.77,87.95 180 top
D103  31.43,93.34 180 top
D201  80.64,87.31 90 top
D202  76.2,73.98 0 top
D203  76.2,70.8 0 top
D204  77.47,87.31 90 top
D205  76.2,64.45 0 top
D206  76.2,67.63 0 top
D301  75.56,47.31 0 top
D302  75.56,42.23 0 top
D303  75.56,37.15 0 top
D304  75.56,32.07 0 top
D305  75.56,26.99 0 top
D306  75.56,17.78 0 top
D307  75.56,12.7 0 top
D308  75.56,7.62 0 top
H101  50.16,49.85 270 top
IC101  41.27,52.39 270 top
IC102  46.35,8.57 180 top
IC103  40.32,88.9 180 top
IC104  40.01,19.37 180 top
IC105  33.66,8.57 180 top
IC201  ULN2803  [DIL18']  58.1,63.82 270 top
LED201  94.93,57.47 90 top
LED202  94.93,62.55 90 top
LED203  94.93,67.63 90 top
LED301  87.95,39.37 90 top
LED302  87.95,29.21 90 top
LED303  87.95,19.05 90 top
LED304  87.95,8.89 90 top
LED305  87.95,34.29 90 top
LED306  87.95,24.13 90 top
LED307  87.95,13.97 90 top
LED308  87.95,3.81 90 top
OK101  24.77,52.7 270 top
OK201  75.25,53.66 90 top
OK202  75.25,59.69 90 top
OK301  58.42,38.42 90 top
OK302  58.42,16.51 90 top
QG101  25.08,35.88 270 top
R101  24.77,71.44 180 top
R102  24.77,74.3 180 top
R103  24.77,68.58 180 top
R104  24.77,62.87 180 top
R105  24.77,65.72 180 top
R106  24.77,48.26 180 top
R107  40.64,84.14 0 top
R108  40.64,81.28 180 top
R109  24.77,57.15 0 top
R201  68.26,68.9 270 top
R202  65.41,68.9 270 top
REL201  64.77,80.96 0 top
REL202  64.77,91.44 0 top
RN301  66.36,38.42 90 top
RN302  66.36,16.51 90 top
SV101  22.86,13.97 270 top
V101  24.77,86.36 180 top
X101  5.08,10.48 270 top
X102  5.08,30.48 270 top
X201  95.57,90.81 270 top
X202  95.57,76.2 270 top
X301  95.57,21.59 270 top
X302  95.57,48.9 270 top

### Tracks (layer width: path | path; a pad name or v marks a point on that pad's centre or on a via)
0  (via drill 0.3)
  Top 0.406: RN302.2 66.99,10.16 68.26,8.89 70.8,8.89 C307.2 | RN302.4 67.31,15.24 68.58,13.97 70.8,13.97 C306.2 | RN302.6 73.34,20.32 | RN302.8 69.22,28.26 70.8,28.26 C304.2 | RN301.2 67.94,32.07 69.22,33.34 70.8,33.34 C303.2 | RN301.4 67.94,37.15 69.22,38.42 70.8,38.42 C302.2 | RN301.6 67.94,42.23 69.22,43.5 70.8,43.5 C301.2 | RN301.8 67.63,47.31 68.9,48.58 73.03,48.58 73.34,48.9
  Top 0.813: v73.34,49.85 73.34,48.9 73.34,44.45 | 73.34,44.45 73.34,39.69 | 73.34,39.69 73.34,34.29 | 73.34,34.29 73.34,29.53 | 73.34,29.53 73.34,24.77 | 73.34,24.77 73.03,24.45 C305.2 | C304.2 73.34,29.53 | C303.2 73.03,34.61 73.34,34.29 | C302.2 73.34,39.69 | C301.2 73.03,44.77 73.34,44.45 | 73.34,24.77 73.34,20.32 73.34,14.92 | 73.34,14.92 73.34,10.16 | 73.34,10.16 73.34,5.71 72.71,5.08 C308.2 | C307.2 73.34,10.16 | C306.2 73.03,15.24 73.34,14.92
  Bottom 0.813: X302.1 89.53,51.44 87.95,49.85 v73.34,49.85
1-G  (via drill 0.3)
  Top 0.61: v71.75,82.23 v71.75,87.63
  Bottom 0.61: v71.75,82.23 D204.C | REL202.6 v71.75,87.63
1-R  (via drill 0.3)
  Top 0.61: REL202.8 v73.66,90.49
  Bottom 0.61: v73.66,90.49 79.06,90.49 D201.A
1-WIRE
  Top 0.406: IC103.2 40.32,77.47 39.37,76.52 IC101.1
+5V  (via drill 0.3)
  Top 0.61: v51.12,54.93 v51.12,52.07 | LED308.A 87.31,2.54 86.36,3.49 86.36,7.62 | 86.36,7.62 86.36,12.38 | 86.36,12.38 86.36,17.78 | 86.36,17.78 86.36,22.54 | 86.36,22.54 86.36,27.94 | 86.36,38.1 86.36,52.07 90.49,56.2 LED201.A | LED304.A 86.36,7.62 | LED307.A 86.68,12.7 86.36,12.38 | LED303.A 86.36,17.78 | LED306.A 86.68,22.86 86.36,22.54 | LED302.A 86.36,27.94 | 86.36,27.94 86.36,33.02 | LED305.A 86.36,33.02 | 86.36,33.02 86.36,38.1 | 86.36,38.1 LED301.A | REL202.9 74.93,95.25 75.25,94.93 v75.25,92.71 75.25,85.09 74.93,84.77 REL201.9
  Top 0.813: v31.11,24.77 31.11,20 28.26,17.14 v28.26,16.51 v28.26,12.7 v28.26,1.91 23.81,1.91 23.18,2.54 C103.1 | v47.31,94.3 46.67,93.66 46.67,92.27 C104.+ 45.21,90.81 38.42,90.81 37.78,90.17 IC103.3 | IC102.3 45.09,9.84 47.62,7.3 IC102.7
  Bottom 0.406: R103.2 18.1,68.58 | R105.2 18.41,65.72 18.1,66.04
  Bottom 0.61: IC101.10 45.09,53.66 46.35,54.93 v51.12,54.93 | IC101.30 50.16,51.12 v51.12,52.07 64.45,52.07 66.04,50.48 72.07,50.48 72.71,51.12 85.41,51.12 90.49,56.2 LED201.A | v47.31,94.3 54.29,94.3 55.88,92.71 v75.25,92.71
  Bottom 0.813: v28.26,1.91 47.94,1.91 48.9,2.86 48.9,4.76 | IC101.10 32.38,53.66 31.43,52.7 31.43,46.04 QG101.14 27.3,43.5 | v28.26,12.7 28.26,10.79 28.89,10.16 31.75,10.16 32.38,10.79 IC105.3 | v31.11,24.77 30.48,25.4 29.53,25.4 27.3,27.62 27.3,43.5 | 48.9,4.76 IC102.7 | IC102.8 48.9,4.76 | IC104.18 IC104.17 45.09,13.02 IC102.3 | 27.3,43.5 27.3,48.58 26.67,49.21 26.67,55.56 25.08,57.15 R109.1 R104.2 18.1,64.45 18.1,66.04 18.1,68.58 18.1,83.19 18.73,83.82 V101.OUT 22.23,85.72 26.35,89.85 31.75,89.85 C105.1 37.47,88.58 IC103.3 | SV101.2 v28.26,16.51
  pour Top: 17.14,76.83 17.14,91.76 42.23,91.76 42.86,92.39 42.86,94.61 43.81,95.57 53.02,95.57 53.02,79.38 32.7,79.38 31.75,78.42 31.75,77.15 30.8,76.2 17.78,76.2
+18V  (via drill 0.3)
  Top 0.406: C106.1 34.61,83.19 R107.1 35.56,92.71 36.2,93.34 D103.C
  Top 0.61: C202.1 IC201.10 57.15,53.66 56.52,54.29 56.52,77.15 | REL201.2 56.52,77.15 | REL202.2 REL202.1 53.98,87.63 | 56.52,77.15 REL201.1 54.29,77.15 53.98,77.47 53.98,87.63 | v53.98,97.79 53.98,87.63
  Top 0.813: v17.14,11.43 17.14,12.06 | 17.14,12.06 v17.14,12.7 | X101.6 17.08,12 17.14,12.06 | X102.6 16.9,32
  Top 1.016: 16.9,32 17.14,31.76 v17.14,31.43 v17.14,32.7
  Bottom 0.61: D103.C 40.32,93.34 41.59,94.61 41.59,96.84 42.55,97.79 v53.98,97.79
  Bottom 0.813: v17.14,11.43 v17.14,12.7 v17.14,31.43 v17.14,32.7 17.14,58.74 14.29,61.59 14.29,82.87 19.37,87.95 D102.A 21.59,87.95 25.08,91.44 27.3,91.44 29.21,93.34 D103.C
/CS-MBC  (via drill 0.3)
  Top 0.406: IC104.16 45.09,19.68 46.35,20.95 46.35,25.72 46.04,26.04 v46.04,66.36
  Bottom 0.406: R105.1 30.48,66.36 IC101.5 v46.04,66.36
/CS-MEM  (via drill 0.3)
  Top 0.406: v35.56,70.17 v35.56,62.55 35.56,27.3 33.66,25.4 v33.66,10.48
  Bottom 0.406: IC101.38 41.59,71.44 40.32,70.17 v35.56,70.17 | R104.1 31.11,62.87 31.43,62.55 v35.56,62.55 | v33.66,10.48 49.53,10.48 50.16,11.11 IC102.1
/RES  (via drill 0.3)
  Top 0.406: v44.13,56.2 44.13,25.72 43.81,25.4 v43.81,19.37 | C102.1 26.04,67.94 26.67,68.58 R103.1 | SV101.5 22.86,12.7 26.04,12.7 26.35,13.02 26.35,18.41 v27.3,19.37
  Bottom 0.406: IC101.37 45.09,68.9 43.81,67.63 30.8,67.63 R103.1 | v44.13,56.2 IC101.9 32.07,56.2 31.43,56.83 31.43,58.74 30.16,60.01 C102.1 | v27.3,19.37 v43.81,19.37
AREF  (via drill 0.3)
  Top 0.406: C101.1 52.39,55.56 v52.07,55.88
  Bottom 0.406: v52.07,55.88 51.75,56.2 IC101.32
BRAUN
  Top 0.61: X201.1 93.34,95.89 92.08,94.61 92.08,80.01 93.34,78.74 X202.1
CAN-H  (via drill 0.3)
  Top 0.406: X101.8 12.32,14.03 v12.38,13.97 | v12.38,33.97 9.46,33.97 X102.8 | v12.38,28.89 v18.73,28.89 | v18.73,45.09 v25.4,45.09 | v25.4,53.98 OK101.4
  Bottom 0.406: IC105.7 34.92,7.62 34.61,7.94 13.02,7.94 12.38,8.57 v12.38,13.97 v12.38,28.89 v12.38,33.97 | v18.73,28.89 v18.73,45.09 | v25.4,45.09 v25.4,53.98
CAN-L  (via drill 0.3)
  Top 0.406: X101.7 7.62,14.29 8.57,15.24 v11.43,15.24 | v11.43,35.24 7.94,35.24 7.62,34.92 X102.7 | v11.43,27.62 v19.68,27.62
  Bottom 0.406: IC105.6 32.38,6.99 32.07,7.3 12.06,7.3 11.43,7.94 v11.43,15.24 v11.43,27.62 v11.43,35.24 | v19.68,27.62 R106.2
GND  (via drill 0.3)
  Top 0.61: REL202.11 69.85,95.25 70.17,94.93 v70.17,91.76 70.17,85.09 69.85,84.77 REL201.11 | OK202.3 72.07,60.96 72.71,60.33 72.71,55.56 72.07,54.93 OK201.3 | C202.2 60.01,50.48 61.59,48.9 63.82,48.9 64.45,49.53 64.45,54.29 65.09,54.93 C201.2
  Top 0.813: 7.3,62.23 16.83,62.23 17.46,61.59 17.46,60.01 | 7.88,43.76 arc90 7.94,43.81 | 17.46,60.01 17.46,52.07 18.1,51.44 OK101.2 21.59,51.44 23.18,49.85 31.43,49.85 32.7,51.12 IC101.11 | C102.2 17.46,60.01 | C101.2 54.93,47.62 OK301.9 52.07,47.31 51.75,46.99 51.75,42.23 | 51.75,42.23 51.75,37.15 | 51.75,37.15 51.75,32.38 | 51.75,32.38 51.75,25.08 | 51.75,25.08 51.75,20 | 51.75,20 51.75,14.92 | 51.75,14.92 51.75,11.11 52.7,10.16 OK302.15 | OK302.13 52.07,15.24 51.75,14.92 | OK302.11 52.07,20.32 51.75,20 | OK302.9 52.07,25.4 51.75,25.08 | OK301.15 52.07,32.07 51.75,32.38 | OK301.13 51.75,37.15 | OK301.11 51.75,42.23 | C101.2 54.93,53.02 IC201.9 | C101.2 C202.2 | IC105.2 v34.92,9.21 | IC105.8 v37.47,9.21 | IC102.4 v42.55,9.21 | v24.13,8.89 SV101.6 | C103.2 v25.72,8.89
  Top 1.016: 8.57,79.69 14.29,79.69 21.27,86.68 23.81,86.68 24.77,85.72 V101.GND | D101.K 8.57,79.69 | 8.57,79.69 8.57,76.2 7.3,74.93 7.3,62.23 7.3,44.45 7.94,43.81 8.57,43.18 | 8.57,43.18 21.27,30.48 QG101.7 | 8.57,79.69 8.57,82.55 6.67,84.45 6.67,89.66 CON101.2 | X102.S@1 8.51,43.12 8.57,43.18
  Top 1.27: IC104.9 29.84,23.5 25.08,28.26 QG101.7
  Bottom 0.406: X101.S@2 8.41,2.38 8.26,2.22
  Bottom 0.61: 50.16,91.95 C104.- 50.35,91.76 v70.17,91.76 | C201.2 OK201.3 | OK202.3 73.03,62.55 83.5,62.55 84.77,63.82 LED202.K 96.52,63.82 97.16,64.45 97.16,68.26 96.52,68.9 LED203.K
  Bottom 0.813: IC101.11 44.13,51.12 46.67,53.66 IC101.31 IC201.9 | 8.26,2.22 8.26,1.91 7.62,1.27 2.86,1.27 2.22,1.91 2.22,11.11 | 2.22,11.11 2.22,20.32 | 2.22,20.32 2.22,28.89 | 2.22,28.89 2.22,38.73 2.86,39.37 7.94,39.37 8.57,38.73 8.57,38.65 X102.S@1 | X101.S@1 X102.S@2 8.57,22.31 8.57,20.32 2.22,20.32 | 2.22,28.89 2.29,28.96 X102.3 7.62,30.16 | X102.5 7.62,30.16 | X102.4 7.81,29.97 7.62,30.16 | 2.22,11.11 2.35,10.99 X101.5 8.06,10.99 8.89,10.16 9.21,10.16 X101.4 | OK302.15 54.45,10.32 52.55,10.32 51.44,9.21 v42.55,9.21 v37.47,9.21 v34.92,9.21 33.02,9.21 32.7,8.89 v25.72,8.89 v24.13,8.89
  pour Bottom: 17.78,91.44 41.91,91.44 42.86,92.39 42.86,94.61 43.81,95.57 53.02,95.57 53.02,79.38 32.7,79.38 31.75,78.42 31.75,77.15 30.8,76.2 17.78,76.2 17.14,76.83 17.14,90.81
GRAU  (via drill 0.3)
  Top 0.61: v61.91,89.53 61.91,82.87 62.87,81.92 62.87,77.79 REL201.4
  Bottom 0.61: v61.91,89.53 81.28,89.53 85.41,93.66 97.16,93.66 98.11,92.71 98.11,86.68 97.16,85.72 X201.3
GRüN  (via drill 0.3)
  Top 0.61: v75.25,83.5 75.25,82.55 73.66,80.96 73.66,79.69 | 73.66,79.69 REL201.8 | v69.53,82.23 69.53,79.69 73.66,79.69
  Bottom 0.61: X201.2 85.09,90.81 81.92,87.63 77.47,87.63 75.25,85.41 v75.25,83.5 | REL202.4 65.41,87.63 66.36,86.68 66.36,82.87 66.99,82.23 v69.53,82.23
I00  (via drill 0.3)
  Top 0.305: v46.99,30.8 v46.99,44.77
  Bottom 0.305: IC101.22 v46.99,30.8 | v46.99,44.77 OK301.10
  Bottom 0.406: OK301.10 60.01,44.77 61.28,43.5 76.52,43.5 79.38,40.64 LED301.K
I01  (via drill 0.3)
  Top 0.305: v56.2,33.34 v56.2,39.69
  Bottom 0.305: IC101.23 v56.2,33.34
  Bottom 0.406: OK301.12 v56.2,39.69 60.01,39.69 61.28,38.42 76.52,38.42 79.38,35.56 LED305.K
I02
  Bottom 0.305: IC101.24 50.8,35.88 52.07,34.61 OK301.14
  Bottom 0.406: OK301.14 60.01,34.61 61.28,33.34 76.52,33.34 79.38,30.48 LED302.K
I03  (via drill 0.3)
  Top 0.305: v57.15,38.42 v57.15,29.53
  Bottom 0.305: IC101.25 v57.15,38.42
  Bottom 0.406: OK301.16 v57.15,29.53 60.01,29.53 61.28,28.26 76.83,28.26 79.69,25.4 LED306.K
I04  (via drill 0.3)
  Top 0.305: v58.1,40.96 v58.1,22.86
  Bottom 0.305: IC101.26 v58.1,40.96
  Bottom 0.406: OK302.10 v58.1,22.86 59.05,22.86 60.33,24.13 67.31,24.13 68.9,25.72 78.11,25.72 83.5,20.32 LED303.K
I05  (via drill 0.3)
  Top 0.305: v59.05,43.5 v59.05,17.78
  Bottom 0.305: IC101.27 v59.05,43.5
  Bottom 0.406: OK302.12 v59.05,17.78 60.01,17.78 61.28,16.51 83.82,16.51 85.09,15.24 LED307.K
I06  (via drill 0.3)
  Top 0.305: v60.01,46.04 v60.01,12.38
  Bottom 0.305: IC101.28 v60.01,46.04
  Bottom 0.406: OK302.14 59.69,12.7 v60.01,12.38 60.96,11.43 83.82,11.43 85.09,10.16 LED304.K
I07  (via drill 0.3)
  Top 0.305: v60.96,48.26 v60.96,6.67
  Bottom 0.305: IC101.29 55.56,48.58 55.88,48.26 v60.96,48.26
  Bottom 0.406: OK302.16 60.01,7.62 v60.96,6.67 61.28,6.35 83.5,6.35 84.77,5.08 LED308.K
IMP-1-G  (via drill 0.3)
  Top 0.61: IC201.15 IC201.16 63.5,68.9 63.82,69.22 63.82,74.61 65.41,76.2 v65.41,82.23 | v58.42,82.23 REL201.15
  Bottom 0.61: v65.41,82.23 v58.42,82.23
IMP-1-R  (via drill 0.3)
  Top 0.61: IC201.17 IC201.18 v61.91,81.28 | v55.88,81.28 REL201.16
  Bottom 0.61: v61.91,81.28 v55.88,81.28
IMP-2-G
  Top 0.61: IC201.11 IC201.12 58.74,58.74 58.42,59.05 58.42,74.3 60.01,75.88 60.01,94.93 59.69,95.25 REL202.15
IMP-2-R  (via drill 0.3)
  Top 0.61: IC201.13 IC201.14 60.01,63.82 59.69,64.14 59.69,74.3 60.96,75.56 v60.96,93.66
  Bottom 0.61: v60.96,93.66 56.52,93.66 55.88,94.3 REL202.16
L  (via drill 0.3)
  Top 0.61: OK201.2 OK202.1 82.55,58.42 83.5,59.37 83.5,65.41 D206.A | v74.93,70.8 v78.11,67.63
  Bottom 0.61: D203.C v74.93,70.8 | v78.11,67.63 D206.A 87.31,73.66 X202.2
LED-G
  Top 0.406: R102.1 32.7,74.3 33.02,73.98 IC101.2
LED-R
  Bottom 0.406: IC101.4 32.38,68.9 R101.1
MISO  (via drill 0.3)
  Top 0.406: IC102.2 47.62,12.7 46.35,13.97 v46.35,17.46 | v39.37,61.28 39.37,27.3 41.27,25.4 v41.27,17.46
  Bottom 0.406: SV101.1 22.86,17.78 29.84,17.78 30.16,17.46 v41.27,17.46 42.55,17.46 | 42.55,17.46 IC104.15 | v46.35,17.46 42.55,17.46 | IC101.7 v39.37,61.28
MOSI  (via drill 0.3)
  Top 0.406: v38.42,63.82 38.42,26.99 38.73,26.67 v38.73,21.27 38.73,15.56 | SV101.4 25.08,13.97 25.4,14.29 25.4,19.05 v27.62,21.27 | 38.73,15.56 38.73,13.97 39.69,13.02 39.69,5.4 40.32,4.76 IC102.5 | IC104.14 38.73,15.56
  Bottom 0.406: IC101.6 v38.42,63.82 | v27.62,21.27 v38.73,21.27
N$1  (via drill 0.3)
  Top 0.406: IC105.1 37.78,12.38 38.73,11.43 v38.73,7.62 | v48.9,7.62 48.9,19.68 50.16,20.95 IC104.1
  Bottom 0.406: v38.73,7.62 v48.9,7.62
N$2  (via drill 0.3)
  Top 0.406: IC105.4 29.84,12.7 31.11,13.97 31.11,17.78 32.07,18.73 32.07,20 v32.38,20.32 | v47.62,20.32 IC104.2
  Bottom 0.406: v32.38,20.32 v47.62,20.32
N$3
  Bottom 0.406: OK101.3 28.57,50.48 29.84,49.21 R106.1
N$4  (via drill 0.3)
  Top 0.61: v74.93,73.98 v78.11,70.8
  Bottom 0.61: D202.C v74.93,73.98 | v78.11,70.8 D203.A
N$5  (via drill 0.3)
  Top 0.406: OK101.1 21.59,53.98 24.77,57.15 R109.2 | X101.3 6.6,8.95 6.35,9.21 6.35,14.29 8.26,16.19 18.1,16.19 18.73,16.83 18.73,22.86 v22.54,26.67
  Bottom 0.406: v22.54,26.67 22.54,52.39 OK101.1
N$6
  Bottom 0.813: D102.C 28.57,87.95 27.3,86.68 V101.IN 27.3,80.64 29.53,78.42 47.31,78.42 48.9,80.01 C107.+
N$7  (via drill 0.3)
  Top 0.61: v74.93,67.63 v78.11,64.45
  Bottom 0.61: D206.C v74.93,67.63 | v78.11,64.45 D205.A
N$8  (via drill 0.3)
  Top 0.406: v65.41,60.33 R202.2
  Bottom 0.406: OK202.2 73.98,60.96 72.71,59.69 66.04,59.69 v65.41,60.33
N$9  (via drill 0.3)
  Top 0.406: R101.2 v12.7,71.44
  Bottom 0.406: v12.7,71.44 6.99,77.15 D101.AR
N$10  (via drill 0.3)
  Top 0.406: v68.58,53.66 68.58,63.5 R201.2
  Bottom 0.406: OK201.1 77.79,53.66 v68.58,53.66
N$11
  Bottom 0.406: D301.A 87,47.31 X301.1
N$12
  Top 0.406: D301.C 70.48,45.72 C301.1 68.26,43.5 64.77,43.5 63.5,44.77 OK301.7
N$13  (via drill 0.3)
  Top 0.406: R102.2 v11.75,74.3
  Bottom 0.406: v11.75,74.3 11.75,76.52 6.03,82.23 D101.AG
N$14
  Top 0.406: D302.C 70.48,40.64 C302.1 68.26,38.42 64.77,38.42 63.5,39.69 OK301.5
N$15
  Top 0.406: D303.C 70.48,35.56 C303.1 68.26,33.34 64.77,33.34 63.5,34.61 OK301.3
N$16
  Bottom 0.406: D302.A 89.53,42.23 91.44,40.32 91.44,37.78 X301.2
N$17
  Bottom 0.406: D303.A 85.41,37.15 85.72,36.83 89.22,36.83 92.08,33.97 92.08,32.07 X301.3
N$18
  Top 0.406: D304.C 70.48,30.48 C304.1 68.26,28.26 64.77,28.26 63.5,29.53 OK301.1
N$19
  Bottom 0.406: D304.A 85.41,32.07 85.72,31.75 89.85,31.75 92.39,29.21 92.39,25.4 93.66,24.13 X301.4
N$20
  Top 0.406: D305.C 70.48,25.4 C305.1 69.53,22.86 68.26,21.59 64.77,21.59 63.5,22.86 OK302.7
N$21
  Top 0.406: D306.C 70.48,16.19 C306.1 68.26,16.51 64.77,16.51 63.5,17.78 OK302.5
N$22
  Top 0.406: D307.C 70.48,11.11 C307.1 68.26,11.43 64.77,11.43 63.5,12.7 OK302.3
N$23
  Top 0.406: D308.C 70.48,6.03 C308.1 68.58,6.03 65.09,6.03 63.5,7.62 OK302.1
N$24
  Bottom 0.406: D305.A 85.41,26.99 85.72,26.67 90.49,26.67 91.12,26.04 91.12,21.27 93.34,19.05 X301.5
N$25
  Bottom 0.406: D306.A 84.14,17.78 85.41,16.51 92.39,16.51 X301.6
N$26
  Bottom 0.406: D308.A 84.14,7.62 85.41,6.35 92.39,6.35 X301.8
N$27
  Bottom 0.406: D307.A 84.14,12.7 85.41,11.43 92.39,11.43 X301.7
N$42
  Top 0.406: OK302.2 63.18,10.16 65.72,7.62 RN302.1
N$43
  Top 0.406: OK302.4 63.18,15.24 65.72,12.7 RN302.3
N$44
  Top 0.406: OK302.6 63.18,20.32 65.72,17.78 RN302.5
N$45
  Top 0.406: OK302.8 63.18,25.4 65.72,22.86 RN302.7
N$46
  Top 0.406: OK301.2 63.18,32.07 65.72,29.53 RN301.1
N$48
  Top 0.406: OK301.4 63.18,37.15 65.72,34.61 RN301.3
N$64
  Top 0.406: OK301.6 63.18,42.23 65.72,39.69 RN301.5
N$65
  Top 0.406: OK301.8 63.18,47.31 65.72,44.77 RN301.7
P00  (via drill 0.3)
  Top 0.406: v43.18,43.5 v43.18,72.71
  Top 0.61: IC201.2 IC201.1
  Bottom 0.406: IC101.14 v43.18,43.5 | v43.18,72.71 50.8,72.71 52.07,71.44 IC201.2
P01  (via drill 0.3)
  Top 0.406: v42.23,40.96 v42.23,70.17
  Top 0.61: IC201.4 IC201.3
  Bottom 0.406: v42.23,70.17 50.8,70.17 52.07,68.9 IC201.3 | IC101.15 v42.23,40.96
P02  (via drill 0.3)
  Top 0.406: v41.27,38.42 v41.27,65.09
  Top 0.61: IC201.5 IC201.6
  Bottom 0.406: v41.27,65.09 50.8,65.09 52.07,63.82 IC201.5 | IC101.16 v41.27,38.42
P03  (via drill 0.3)
  Top 0.406: v40.32,35.88 v40.32,57.47
  Top 0.61: IC201.8 IC201.7
  Bottom 0.406: v40.32,57.47 52.39,57.47 53.66,56.2 IC201.8 | IC101.17 v40.32,35.88
P04  (via drill 0.3)
  Top 0.406: v45.09,33.34 v45.09,60.01 | v74.3,58.42 v74.3,52.39
  Bottom 0.406: IC101.18 v45.09,33.34 | v45.09,60.01 64.14,60.01 66.04,58.42 OK202.4 v74.3,58.42 | v74.3,52.39 OK201.4 C201.1
PLUGGED  (via drill 0.3)
  Top 0.406: v13.02,72.71 35.24,72.71 v35.56,73.03
  Bottom 0.406: IC101.39 36.51,73.98 v35.56,73.03 | CON101.3 10.65,79.84 13.02,77.47 v13.02,72.71
Q-CLK  (via drill 0.3)
  Top 0.406: IC104.8 32.38,25.08 30.8,26.67 v30.8,28.26 QG101.8
  Bottom 0.406: IC101.13 30.8,43.18 v30.8,28.26
SCH-1-G  (via drill 0.3)
  Top 0.61: v66.36,90.81 66.36,75.25 65.41,74.3 R202.1 65.41,70.17 D205.C
  Bottom 0.61: v66.36,90.81 70.8,90.81 71.44,91.44 76.52,91.44 D204.A
SCH-1-R
  Top 0.61: D201.C 80.64,81.92 81.28,81.28 D202.A
  Bottom 0.61: R201.1 69.85,72.39 79.69,72.39 D202.A
SCK  (via drill 0.3)
  Top 0.406: v36.51,58.74 36.51,26.04 36.2,25.72 36.2,20 v37.47,18.41 IC104.13 37.47,14.92 36.2,13.65 36.2,3.49 36.83,2.86 44.45,2.86 45.09,3.49 IC102.6
  Bottom 0.406: IC101.8 v36.51,58.74 | SV101.3 20.95,13.97 20,14.92 20,17.46 20.95,18.41 v37.47,18.41
SEL1  (via drill 0.3)
  Top 0.406: REL201.13 63.5,84.14 63.82,83.82 v63.82,81.28 | v72.71,75.25 v72.71,66.04
  Bottom 0.406: IC101.36 51.12,66.36 52.39,65.09 68.58,65.09 69.53,66.04 v72.71,66.04 94.61,66.04 LED203.A | v63.82,81.28 71.75,81.28 72.07,80.96 72.07,75.88 v72.71,75.25
SEL2  (via drill 0.3)
  Top 0.406: v57.47,57.47 v57.47,62.55 | REL202.13 v63.5,90.81 | v53.02,90.81 53.02,75.88 51.75,74.61 51.75,65.41 50.16,63.82 IC101.35
  Top 0.61: LED201.K LED202.A
  Bottom 0.406: LED202.A 88.27,61.28 83.82,56.83 64.77,56.83 64.14,57.47 v57.47,57.47 | v57.47,62.55 51.75,62.55 50.48,63.82 IC101.35 | v63.5,90.81 v53.02,90.81
SPG
  Top 0.406: R107.2 R108.1 45.72,77.15 46.35,76.52 IC101.40
V-NETZTEIL1
  Top 1.016: CON101.1 19.05,90.49 21.91,93.34 D103.A

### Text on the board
Bottom: MBCAN-Projekt | (c) Dr.-Ing. Th. Wiesner | 20.02.2024 | mbc86.brd | bottom
tNames: HW: 24.02.20 | 0 | Gn | 7294 | Gr | +18V | DC | 0 | Trafo | (c) Dr.-Ing. Th. Wiesner | MBCAN-Projekt | L | On | > | Status 7294 | < | 0 | Gleis | B | 1 | IN | 2 | 3 | 4 | 5 | OUT | 6 | 7 | 8 | mbc-86 | +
